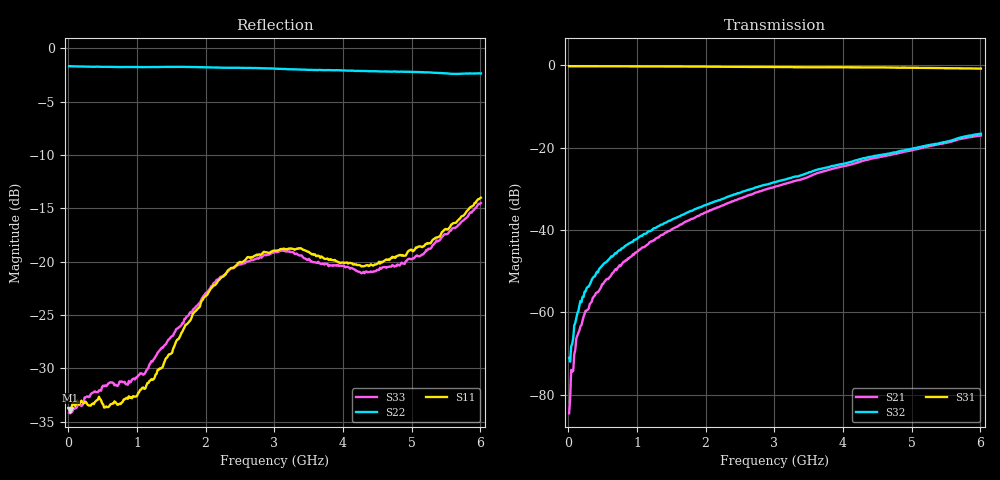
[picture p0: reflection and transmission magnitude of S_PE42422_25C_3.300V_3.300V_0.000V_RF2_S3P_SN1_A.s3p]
! Device ID: PE42422
! Serial: 1
! Insertion: A
! Temp: 25C
! VDD: 3.300
! Control_Hi: 3.300
! Control_Lo: 0.000
! Logic State: RF2
! Port 1: RFC
! Port 2: RF1
! Port 3: RF2
! ThroughPath:3-1
! V1 = 0.00
! V2 = 0.00
! V3 = 0.00
! V4 = 0.00
! IDD: 1.025153e-04
#  Hz  S  RI  R  50
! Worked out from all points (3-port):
!   401 points, 10 MHz to 6.01 GHz, reference 50 ohm
!   strongest paths, dB at 10 MHz, 1.51 GHz, 3.01 GHz, 4.51 GHz, 6.01 GHz:
!     S31: -0.2, -0.3, -0.4, -0.5, -0.8
!     S32: -71.1, -37.4, -28.4, -21.9, -16.6
!     S21: -84.5, -39.8, -29.5, -22.3, -17.0
!   lowest |S11| = -33.9 dB at 25 MHz (marker M1), VSWR 1.04, Z = 52.1 + j0.0736 ohm
!   |S11| at or under -10 dB: start of sweep to end of sweep
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1e7  0.0204 9.14e-05  -4.2e-05 -5.05e-05  0.9763 -0.00167
     -3.89e-05 -4.52e-05  -0.8245 0.00224  7.2e-05 -0.000176
     0.9766 -0.00155  0.000188 0.000208  0.0195 -0.000171
2.5e7  0.0202 0.000707  1.93e-05 0.000124  0.9767 -0.00407
       7.03e-05 5.38e-05  -0.8246 0.00579  0.000107 0.000158
       0.9764 -0.00403  -2.98e-05 0.00025  0.0194 0.000958
1.15e8  0.0218 0.00159  -5.17e-05 0.000505  0.9756 -0.0169
        -1.61e-05 0.000484  -0.8217 0.0255  0.000131 0.000824
        0.9754 -0.0169  -2e-05 0.000849  0.0205 0.0021
2.35e8  0.0218 0.00145  -0.000116 0.00091  0.9743 -0.0341
        -0.000178 0.000942  -0.8185 0.0503  -3e-05 0.00168
        0.9746 -0.0343  -4.63e-05 0.00179  0.023 0.00134
7.15e8  0.0209 -0.00417  -0.00153 0.00301  0.9677 -0.1015
        -0.00161 0.00307  -0.806 0.1353  -0.000927 0.00531
        0.968 -0.1012  -0.00102 0.00537  0.0257 -0.00472
1.66e9  -0.000468 -0.0469  -0.00762 0.00954  0.9397 -0.2313
        -0.00735 0.00936  -0.7728 0.2693  -0.00565 0.0143
        0.94 -0.2309  -0.0056 0.0142  0.0176 -0.0485
2.35e9  -0.0278 -0.0878  -0.0136 0.0168  0.9053 -0.3216
        -0.0137 0.0168  -0.7316 0.3499  -0.0105 0.0238
        0.9043 -0.3207  -0.0105 0.0237  -0.00414 -0.0918
3.01e9  -0.047 -0.1024  -0.0199 0.0271  0.8654 -0.4026
        -0.0201 0.0268  -0.6778 0.4314  -0.0148 0.0349
        0.8649 -0.4027  -0.0147 0.0351  -0.0257 -0.1079
4.45e9  -0.0623 -0.0731  -0.0354 0.0658  0.7485 -0.5767
        -0.0354 0.0658  -0.4795 0.6166  -0.0227 0.0756
        0.7478 -0.5765  -0.0228 0.0759  -0.0448 -0.0782
6.01e9  -0.1911 -0.0566  -0.0255 0.1391  0.5367 -0.7398
        -0.0244 0.1385  -0.2494 0.7208  -0.00951 0.1472
        0.5347 -0.7388  -0.011 0.1473  -0.144 -0.1213
